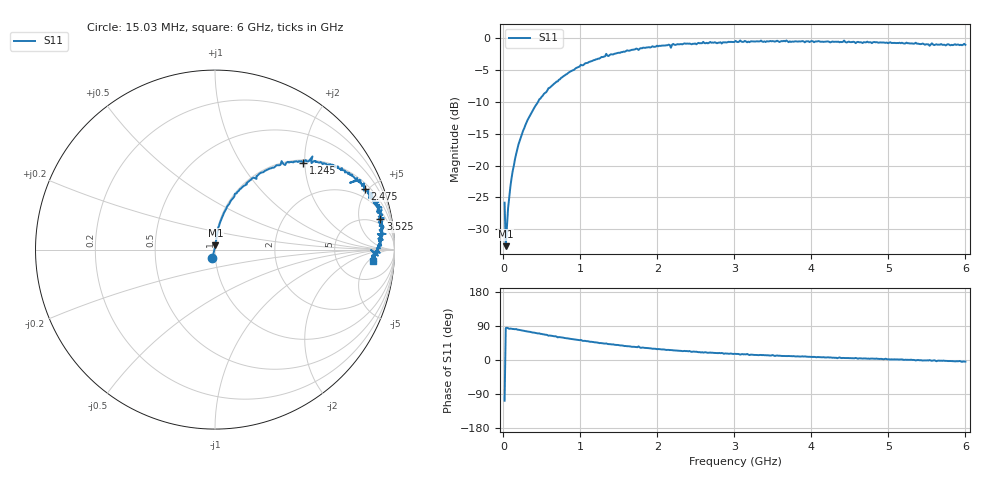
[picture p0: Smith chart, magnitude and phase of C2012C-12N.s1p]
!	Network	Analyzer	HP8753E.07.74:	Oct	30	2002	Serial	No.	JP38451487
!	Hewlett-Packard
!	7	Sep	2009	10:44:24
!	Frequency	S11
#	HZ	S	RI	R	50
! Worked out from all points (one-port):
!   400 points, 15.03 MHz to 6 GHz, reference 50 ohm
!   lowest |S11| = -32.6 dB at 30.03 MHz (marker M1), VSWR 1.05, Z = 50.2 + j2.33 ohm
!   |S11| at or under -10 dB: start of sweep to 450.2 MHz
!   S11 on the Smith chart (normalised r, x): 15.03 MHz: 0.97, -0.09; 1.245 GHz: 1.07, +1.96; 2.475 GHz: 1.33, +4.74; 3.525 GHz: 3, +10; 6 GHz: 12, -7
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1.502992e7  -0.0153 -0.0488
3.002985e7  0.00235 0.0232
6.00297e7  0.00485 0.0459
9.002955e7  0.00838 0.0678
1.500292e8  0.0169 0.111
2.10029e8  0.0289 0.153
3.150284e8  0.0585 0.221
4.650277e8  0.111 0.311
7.650262e8  0.25 0.425
1.005025e9  0.371 0.493
1.245024e9  0.491 0.483
1.335023e9  0.543 0.519
1.515022e9  0.599 0.476
1.99502e9  0.765 0.415
2.160019e9  0.792 0.389
2.175019e9  0.752 0.372
2.205019e9  0.811 0.387
2.265019e9  0.812 0.377
2.475018e9  0.833 0.34
3.015015e9  0.911 0.266
3.165014e9  0.89 0.256
3.195014e9  0.904 0.209
3.495013e9  0.921 0.215
3.525012e9  0.921 0.171
3.765011e9  0.921 0.167
4.515007e9  0.925 0.0799
5.265004e9  0.91 0.00571
6e9  0.882 -0.0645
